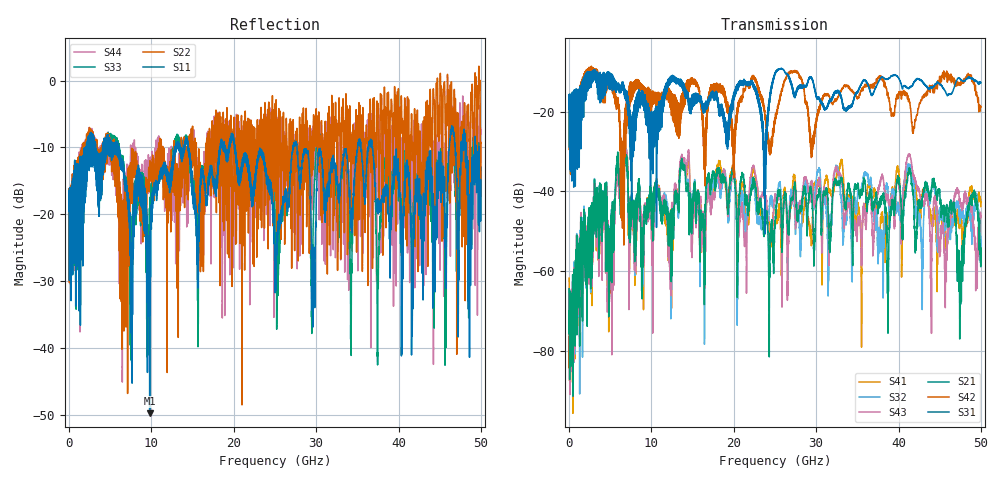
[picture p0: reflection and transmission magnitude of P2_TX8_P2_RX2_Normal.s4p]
!Keysight Technologies,N5225B,MY57041031,A.13.20.10
!Date: Friday, May 31, 2019 11:29:46
!Correction: S11(Full 4 Port(1,2,3,4))
!S12(Full 4 Port(1,2,3,4))
!S13(Full 4 Port(1,2,3,4))
!S14(Full 4 Port(1,2,3,4))
!S21(Full 4 Port(1,2,3,4))
!S22(Full 4 Port(1,2,3,4))
!S23(Full 4 Port(1,2,3,4))
!S24(Full 4 Port(1,2,3,4))
!S31(Full 4 Port(1,2,3,4))
!S32(Full 4 Port(1,2,3,4))
!S33(Full 4 Port(1,2,3,4))
!S34(Full 4 Port(1,2,3,4))
!S41(Full 4 Port(1,2,3,4))
!S42(Full 4 Port(1,2,3,4))
!S43(Full 4 Port(1,2,3,4))
!S44(Full 4 Port(1,2,3,4))
!S4P File: Measurements: <S11,S12,S13,S14>,
!<S21,S22,S23,S24>,
!<S31,S32,S33,S34>,
!<S41,S42,S43,S44>:
# Hz S  dB  R 50.0
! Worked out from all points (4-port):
!   5000 points, 10 MHz to 50 GHz, reference 50 ohm
!   strongest paths, dB at 10 MHz, 12.51 GHz, 25.01 GHz, 37.51 GHz, 50 GHz:
!     S31: -19.3, -11.6, -10.3, -12.8, -12.8
!     S42: -19.4, -15.8, -22.0, -11.5, -18.9
!     S21: -64.4, -44.4, -47.2, -44.9, -54.3
!     S43: -65.7, -42.7, -40.7, -39.1, -46.3
!     S32: -74.0, -43.6, -43.8, -52.4, -52.6
!     S41: -61.8, -44.2, -43.4, -52.8, -43.8
!   lowest |S11| = -49.8 dB at 9.79 GHz (marker M1), VSWR 1.01, Z = 49.9 - j0.321 ohm
!   |S11| at or under -10 dB: 20.17 GHz to 27.18 GHz (7.009 GHz wide, 29.6 % of centre); 27.67 GHz to 35.04 GHz (7.368 GHz wide, 23.5 % of centre); 36.79 GHz to 46.16 GHz (9.373 GHz wide, 22.6 % of centre)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
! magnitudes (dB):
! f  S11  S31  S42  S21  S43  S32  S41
! 10 MHz  -19.6  -19.3  -19.4  -64.4  -65.7  -74.0  -61.8
! 3.23 GHz  -13.5  -11.3  -10.8  -45.0  -47.1  -45.0  -47.0
! 4.89 GHz  -9.4  -12.2  -12.6  -66.9  -61.1  -60.4  -64.0
! 6.46 GHz  -12.3  -13.9  -28.9  -34.5  -33.2  -33.2  -34.6
! 9.79 GHz  -49.8  -26.2  -14.9  -40.1  -41.4  -40.7  -40.6
! 41.25 GHz  -15.7  -14.2  -17.2  -35.1  -30.9  -34.2  -34.1
! 50 GHz  -14.9  -12.8  -18.9  -54.3  -46.3  -52.6  -43.8
